(* Logix 5000 AddOnInstructionDefinition export AOI_spLink; software revision 36.00 *)

TYPE DUT_NDSN_spLink :   // UDDT that holds the Cyclic and ACyclic data for the SpectraLink.
STRUCT
   b_r_LostComm : BOOL;
   b_r_PLC_CommReadOnly : BOOL;
   b_r_SystemReady : BOOL;   // Pattern Status Word 0 Bit 0
   b_r_Fault : BOOL;   // Pattern Status Word 0 Bit 1
   b_r_Alert : BOOL;   // Pattern Status Word 0 Bit 2
   b_r_Commissioned : BOOL;   // Pattern Status Word 0 Bit 3
   b_r_RecipeModified : BOOL;   // Pattern Status Word 0 Bit 5
   i_r_Recipe : INT;
   i_r_PalletizedCount : INT;
   i_r_PalletizedSkipCount : INT;
   di_r_App_Trig_ProductCount : DINT;
   di_r_FeedCount : DINT;
   di_r_DeliveryCount : DINT;
   st_r_AppStat : DUT_NDSN_spLink_Chan_Status[8];
   st_r_TrigStat : DUT_NDSN_spLink_Trig_Status[8];
   st_r_EncoStat : DUT_NDSN_spLink_Encoder_Status[8];
   i_r_ProductLength : DINT[8];
   i_r_ProdRate : INT;
   i_r_LineSpeed : INT[2];   // m/min units
   i_r_RunupOutput : INT[2];
   b_w_UnitEnable : BOOL;   // Pattern Control Word 0 Bit 0
   b_w_ClearAllAlarms : BOOL;   // Clear all System Faults and Alerts (Rising Edge).
   b_w_ResetAllCounters : BOOL;   // Reset all counters (rising edge).
   i_w_LoadRecipe : INT;
   i_w_PalletizedCount : INT;   // Write 0 to decrement; 1 to increment; 2 to reset; else does nothing.
   i_w_PalletizedSkipCount : INT;   // Write 0 to decrement; 1 to increment; 2 to reset; else does nothing.
   di_w_App_Trig_ProductCount : DINT;
   di_w_FeedCountReset : DINT;
   di_w_DeliveryCountReset : DINT;
   st_w_AppCtl : DUT_NDSN_spLink_Chan_CTL[8];
   st_rw_BeadAgg : DUT_NDSN_spLink_Bead[8];
   i_rw_RnUpPercentOutP1 : INT[2];
   i_rw_RnUpLineSpdP1 : INT[2];
   i_rw_RnUpPercentOutP2 : INT[2];
   i_rw_RnUpLineSpdP2 : INT[2];
   i_rw_RnUpLowLim : INT[2];
   i_rw_RnUpHighLim : INT[2];
   di_rw_EncoderRes : DINT[2];
   i_rw_TriggerMaskDist : DINT[8];
   i_rw_TriggerChCtl : INT[8];
   i_rw_EncoderChCtl : INT[2];
   i_rw_RandAdjStart : INT[8];
   i_rw_RandAdjEnd : INT[8];
   i_rw_VirtualTriggerSize : DINT[8];
   i_rw_ContStartSpeed : INT[8];
   i_rw_ContStopSpeed : INT[8];
   i_rw_ContKnifeCutDelay : DINT[8];
   i_rw_ContKnifeCutGap : DINT[8];
   di_rw_GTO : DINT[8];
   i_r_ErrorInfo : INT[4];
   i_r_SpecCtl : INT[4];
   i_r_CurrentFault : INT;
END_STRUCT
END_TYPE

TYPE DUT_NDSN_spLink_Bead :
STRUCT
   di_rw_NumOfBeads : DINT;
   di_rw_BeadDelay : DINT[8];   // 1/4 mm
   di_rw_BeadDuration : DINT[8];   // 1/4 mm
   di_rw_mode : DINT;   // 1/4 mm
   di_rw_MaxGunTime : DINT;   // microseconds
   di_rw_LineSpeedActivation : DINT;   // 100th m/min
   di_rw_LineSpeedDeactivation : DINT;   // 100th m/min
   di_rw_Interval : DINT;   // 1/4 mm
   di_rw_AdhesiveSavings : DINT;   // 30%-60%
   di_rw_EcoBeadPattern : DINT;   // 0-40, Illegal values: 0,1,11,20,21,30,31,38,39
END_STRUCT
END_TYPE

TYPE DUT_NDSN_spLink_Chan_CTL :
STRUCT
   b_w_Enable : BOOL;
   b_w_Purge : BOOL;
END_STRUCT
END_TYPE

TYPE DUT_NDSN_spLink_Chan_Status :
STRUCT
   b_r_Enabled : BOOL;
   b_r_Fault : BOOL;
   b_r_Alert : BOOL;
   b_r_Output_Active : BOOL;
   b_r_Installed : BOOL;
END_STRUCT
END_TYPE

TYPE DUT_NDSN_spLink_Encoder_Status :   // SpectraLink Encoder Channel Status
STRUCT
   b_r_Missing : BOOL;
   b_r_Phase_Missing : BOOL;
   b_r_Scaled : BOOL;
   b_r_Fault : BOOL;
   b_r_Alert : BOOL;
   b_r_Installed : BOOL;
END_STRUCT
END_TYPE

TYPE DUT_NDSN_spLink_Rd_Wt :
STRUCT
   i_arr_ReadValue : INT[60];
   i_ReadADI : INT;
   b_ReadDone : BOOL;
   i_arr_WriteValue : INT[60];
   i_WriteADI : INT;
   i_WriteSizeBytes : INT;
   b_WriteEvent : BOOL;
   b_WriteDone : BOOL;
   b_FirstScan : BOOL;
   b_AllowWrites : BOOL;
   b_WriteErr : BOOL;
   b_ReadErr : BOOL;
END_STRUCT
END_TYPE

TYPE DUT_NDSN_spLink_Trig_Status :   // SpectraLink Trigger Channel Status
STRUCT
   b_r_Detected : BOOL;
   b_r_Fault : BOOL;
   b_r_Alert : BOOL;
   b_r_Active : BOOL;
   b_r_Installed : BOOL;
END_STRUCT
END_TYPE

TYPE DUT_spLink_ADI :
STRUCT
   i_ADI : INT;
   i_Size : INT;
END_STRUCT
END_TYPE

ADD_ON_INSTRUCTION AOI_spLink   (* revision 1.0 *)
// AOI to handle the I/O based data (Default Data) and Acyclic Data (low Priority) from the SpectraLink Pattern Controller.
VAR_IN_OUT
   IO_Input : INT[64]; {required}
   IO_Out : INT[64]; {required}
   spLink_HMI : DUT_NDSN_spLink; {required}
   IO_AcycRdWt : DUT_NDSN_spLink_Rd_Wt; {required}
   ReadMsg : MESSAGE; {required}
   WriteMsg : MESSAGE; {required}
   Read_Buffer : INT[100]; {required}
   Write_Buffer : INT[100]; {required}
END_VAR
VAR
   st_ADI_List : DUT_spLink_ADI[40]; {access None}
   tm_Command : FBD_TIMER; {access None}
   tm_Acyc : FBD_TIMER; {access None}
   b_AdhesiveOn : BOOL; {access None}
   b_AdhesiveOff : BOOL; {access None}
   b_Read : BOOL; {access None}
   i_ADI_Range : INT; {access None}
   i_ADI_Size : INT := 20; {access None}
   i_CompareIndex : INT; {access None}
   i_Index : INT; {access None}
   i_Index_Write : INT; {access None}
   i_rwADI_Count : INT := 12; {access None}
   i_rwDataSize : INT := 24; {access None}
   i_Size : INT; {access None}
   i_SizeofStruct : INT := 48; {access None}
   i_ValueIndex : INT; {access None}
   i : INT; {access None}
   i_temp_CPC : INT; {access None}
   arr_WriteIndex : DINT[40]; {access None}
   arr_WriteStartingAddress : DINT[40]; {access None}
   b_AcycWT_Rising : BOOL; {access None}
   arr_HMI : INT[600]; {access None}
   arr_HMI_Buffer : INT[600]; {access None}
   arr_HMI_Compare : INT[600]; {access None}
   b_AcycRD_Rising : BOOL; {access None}
   b_CommandRising : BOOL; {access None}
   tm_PalletizedCount_Reset : FBD_TIMER; {access None}
   b_ResetCurrentPalletizedCount : BOOL; {access None}
   b_ResetCurrentPalletizedSkipCount : BOOL; {access None}
   tm_PalletizedSkipCount_Reset : FBD_TIMER; {access None}
   i_temp_CPSC : INT; {access None}
   i_LoopCnt : INT; {access None}
   b_ResetSelectCount : BOOL; {access None}
   tm_ResetSelectCount : FBD_TIMER := (PRE := 5000); {access None}
   TRUE : BOOL := 1; {access None}
   FALSE : BOOL; {access None}
   tm_ResetFeedCount : FBD_TIMER; {access None}
   tm_ResetDeliveryCount : FBD_TIMER; {access None}
   i_WriteSizeTemp : INT; {access None}
   i_ReadADI_Temp : INT; {access None}
   tm_WriteEvent : FBD_TIMER; {access None}
   b_WriteEventONS : BOOL; {access None}
   i_WritePtr : DINT; {access None}
   Read_Watchdog : FBD_TIMER; {access None}
   Read_Time_Tic : FBD_TIMER; {access None}
   DINT_TEMP : DINT; {access None}
   DINT_Offset : INT; {access Read Only}
END_VAR

ROUTINE Logic   (* structured text *)
   //
   //		SpectraLink Add-On Instruction used to read/write Cyclic (high priority I/O)
   //		and Acyclic (low priority) data.
   //
   //
   //*******************************************************************************
   //	Initialize Code
   //*******************************************************************************
   
   IF IO_AcycRdWt.b_FirstScan THEN
   	i_ADI_Size:= 29;
   	i_rwADI_Count :=26;
   	i_SizeofStruct := 531;
   	i_rwDataSize := 522;
   	i_ADI_Range := 0;
   	i_ValueIndex :=0;
   	i_Index:=0;
   	IO_AcycRdWt.b_FirstScan := 0;		//Reset the FirstScan bit sent to the ADI from the main routine.
   	IO_AcycRdWt.b_AllowWrites := 0;		//Cycle through the full Read Data Set before allowing Writes to occur.  This populates the write compare buffers.
   
   	FOR i := 0 TO i_rwADI_Count DO
   		i_ADI_Range := i_ADI_Range + st_ADI_List[i].i_Size;
   		arr_WriteIndex[i] := i_ADI_Range;					//Index of all Read/Write ADI
   		arr_WriteStartingAddress[i + 1] := i_ADI_Range;		//All Read/Write ADI Starting Address
   	END_FOR;
   
   
   END_IF;
   
   
   
   
   //*******************************************************************************
   //  Start of Cyclic Data Code
   //
   //	The following code handles the I/O data for the High Priority DEFAULT ADIs.
   //*******************************************************************************
   
   // SpectraLink system Status
   spLink_HMI.b_r_SystemReady := IO_Input[0].0;
   spLink_HMI.b_r_Fault := IO_Input[0].1;
   spLink_HMI.b_r_Alert := IO_Input[0].2;
   spLink_HMI.b_r_Commissioned := IO_Input[0].3;
   spLink_HMI.b_r_PLC_CommReadOnly := IO_Input[0].4;
   spLink_HMI.b_r_RecipeModified := IO_Input[0].5;
   
   spLink_HMI.i_r_Recipe := IO_Input[4];
   spLink_HMI.i_r_PalletizedCount := IO_Input[5];
   spLink_HMI.i_r_PalletizedSkipCount := IO_Input[6];
   
   COP(IO_Input[7], spLink_HMI.di_r_App_Trig_ProductCount, 6);
   
   // Copy the Applicator Status Structure Bits from the IO_Inputs
   i_LoopCnt := 0;
   While (i_LoopCnt < 8) DO
   	spLink_HMI.st_r_AppStat[i_LoopCnt].b_r_Enabled := IO_Input[13+i_LoopCnt].0;
   	spLink_HMI.st_r_AppStat[i_LoopCnt].b_r_Fault := IO_Input[13+i_LoopCnt].1;
   	spLink_HMI.st_r_AppStat[i_LoopCnt].b_r_Alert := IO_Input[13+i_LoopCnt].2;
   	spLink_HMI.st_r_AppStat[i_LoopCnt].b_r_Output_Active := IO_Input[13+i_LoopCnt].3;
   	spLink_HMI.st_r_AppStat[i_LoopCnt].b_r_Installed := IO_Input[13+i_LoopCnt].4;
   	i_LoopCnt := i_LoopCnt+1;
   end_while;
   
   // Copy the Trigger Status Structure Bits from the IO_Inputs
   i_LoopCnt := 0;
   While (i_LoopCnt < 8) DO
   	spLink_HMI.st_r_TrigStat[i_LoopCnt].b_r_Detected := IO_Input[21+i_LoopCnt].0;
   	spLink_HMI.st_r_TrigStat[i_LoopCnt].b_r_Fault := IO_Input[21+i_LoopCnt].1;
   	spLink_HMI.st_r_TrigStat[i_LoopCnt].b_r_Alert := IO_Input[21+i_LoopCnt].2;
   	spLink_HMI.st_r_TrigStat[i_LoopCnt].b_r_Active := IO_Input[21+i_LoopCnt].3;
   	i_LoopCnt := i_LoopCnt+1;
   end_while;
   
   // Copy the Encoder Status Structure Bits from the IO_Inputs
   i_LoopCnt := 0;
   While (i_LoopCnt < 2) DO
   	spLink_HMI.st_r_EncoStat[i_LoopCnt].b_r_Missing := IO_Input[29+i_LoopCnt].0;
   	spLink_HMI.st_r_EncoStat[i_LoopCnt].b_r_Phase_Missing := IO_Input[29+i_LoopCnt].1;
   	spLink_HMI.st_r_EncoStat[i_LoopCnt].b_r_Scaled := IO_Input[29+i_LoopCnt].2;
   	spLink_HMI.st_r_EncoStat[i_LoopCnt].b_r_Fault := IO_Input[29+i_LoopCnt].3;
   	spLink_HMI.st_r_EncoStat[i_LoopCnt].b_r_Alert := IO_Input[29+i_LoopCnt].4;
   	i_LoopCnt := i_LoopCnt+1;
   end_while;
   
   
   //******************************************************************************************************************
   //Adjust the Product Length by a factor of 4
   //******************************************************************************************************************
   
   i_LoopCnt := 0;
   While (i_LoopCnt < 8) DO
   	DINT_Offset := i_LoopCnt*2;
   	COP(IO_Input[31+DINT_Offset], DINT_TEMP, 2);
   	spLink_HMI.i_r_ProductLength[i_LoopCnt] := (DINT_TEMP/4);
   	i_LoopCnt := i_LoopCnt+1;
   end_while;
   
   
   COP(IO_Input[47], spLink_HMI.i_r_ProdRate, 1);
   COP(IO_Input[48], spLink_HMI.i_r_LineSpeed[0], 2);
   COP(IO_Input[50], spLink_HMI.i_r_RunupOutput[0], 2);
   
   
   //******************************************************************************************************************
   //Cyclic WRITE Section
   //******************************************************************************************************************
   
   IO_Out[0].0 := spLink_HMI.b_w_UnitEnable;
   IO_Out[2].0 := spLink_HMI.b_w_ClearAllAlarms;
   IO_Out[2].1 := spLink_HMI.b_w_ResetAllCounters;
   
   IO_Out[4] := spLink_HMI.i_w_LoadRecipe;
   
   
   //********************************************************************************************************************************
   //Current Palatized Count & Current Palatized Skip Count     increment (1) or decrement (0);  else = other value     (ADI 16359 Write)
   //********************************************************************************************************************************
   //*********************************************************************
   //PLC logic will set the increment flag (1) or the decrement flag (0) which will generate a 1 second pulse to the spLink.  The
   //command must be set to a "else value" before another increment or decrement can occur.
   //*********************************************************************
   
   IF (spLink_HMI.i_w_PalletizedCount <> i_temp_CPC) AND NOT tm_PalletizedCount_Reset.EN AND NOT b_ResetCurrentPalletizedCount then
   	b_ResetCurrentPalletizedCount := 1;
   	i_temp_CPC := spLink_HMI.i_w_PalletizedCount;
   	tm_PalletizedCount_Reset.Reset := NOT b_ResetCurrentPalletizedCount;
   end_if;
   
   tm_PalletizedCount_Reset.PRE :=2000;
   tm_PalletizedCount_Reset.TimerEnable := b_ResetCurrentPalletizedCount;
   TONR(tm_PalletizedCount_Reset);
   
   If tm_PalletizedCount_Reset.DN then
   	b_ResetCurrentPalletizedCount := 0;
   end_if;
   
   
   IF (tm_PalletizedCount_Reset.EN AND NOT tm_PalletizedCount_Reset.DN AND (i_temp_CPC = 0)) then
   	IO_Out[5] := 0;
   elsif (tm_PalletizedCount_Reset.EN AND NOT tm_PalletizedCount_Reset.DN AND (i_temp_CPC = 1)) then
   	IO_Out[5] := 1;
   else
   	IO_Out[5] := 5;  // anything but a 1 or 0
   end_if;
   
   
   IF (spLink_HMI.i_w_PalletizedSkipCount <> i_temp_CPSC) AND NOT tm_PalletizedSkipCount_Reset.EN AND NOT b_ResetCurrentPalletizedSkipCount then
   	b_ResetCurrentPalletizedSkipCount := 1;
   	i_temp_CPSC := spLink_HMI.i_w_PalletizedSkipCount;
   	tm_PalletizedCount_Reset.Reset := NOT b_ResetCurrentPalletizedSkipCount;
   end_if;
   
   tm_PalletizedSkipCount_Reset.PRE :=2000;
   tm_PalletizedSkipCount_Reset.TimerEnable := b_ResetCurrentPalletizedSkipCount;
   TONR(tm_PalletizedSkipCount_Reset);
   
   IF (tm_PalletizedSkipCount_Reset.EN AND NOT tm_PalletizedSkipCount_Reset.DN AND (i_temp_CPSC = 0)) then
   	IO_Out[6] := 0;
   elsif (tm_PalletizedSkipCount_Reset.EN AND NOT tm_PalletizedSkipCount_Reset.DN AND (i_temp_CPSC = 1)) then
   	IO_Out[6] := 1;
   else
   	IO_Out[6] := 5;  // anything but a 1 or 0
   end_if;
   
   
   If tm_PalletizedSkipCount_Reset.DN then
   	b_ResetCurrentPalletizedSkipCount := 0;
   end_if;
   
   
   //********************************************************************************************************************************
   //Display Select Count, Feed Count and Delivery Count Reset     reset (1) or do nothing (0);        (ADI 16656 Write)
   //********************************************************************************************************************************
   //*********************************************************************
   //PLC logic will set the Reset (1) which will generate a 1 second pulse to the spLink.  The
   //command must be set to a "0" before another Reset can occur.
   //*********************************************************************
   
   
   	tm_ResetSelectCount.PRE := 1000;
   	tm_ResetSelectCount.TimerEnable := spLink_HMI.di_w_App_Trig_ProductCount.0;
   	tm_ResetSelectCount.Reset := NOT spLink_HMI.di_w_App_Trig_ProductCount.0;
   	TONR(tm_ResetSelectCount);
   
   	IF tm_ResetSelectCount.TT then
   		IO_Out[7] := 1;
   	else
   		IO_Out[7] := 0;
   	end_if;
   
   
   	tm_ResetFeedCount.PRE := 1000;
   	tm_ResetFeedCount.TimerEnable := spLink_HMI.di_w_FeedCountReset.0;
   	tm_ResetFeedCount.Reset := NOT spLink_HMI.di_w_FeedCountReset.0;
   	TONR(tm_ResetFeedCount);
   
   	IF tm_ResetFeedCount.TT then
   		IO_Out[9] := 1;
   	else
   		IO_Out[9] := 0;
   	end_if;
   
   
   	tm_ResetDeliveryCount.PRE := 1000;
   	tm_ResetDeliveryCount.TimerEnable := spLink_HMI.di_w_DeliveryCountReset.0;
   	tm_ResetDeliveryCount.Reset := NOT spLink_HMI.di_w_DeliveryCountReset.0;
   	TONR(tm_ResetDeliveryCount);
   
   	IF tm_ResetDeliveryCount.TT then
   		IO_Out[11] := 1;
   	else
   		IO_Out[11] := 0;
   	end_if;
   
   
   //********************************************************************************************************************************
   //Send the Applicator Channel Control Aggregate data to the PC.       (ADI 18675 Write)
   //********************************************************************************************************************************
   
   	i_LoopCnt := 0;
   While (i_LoopCnt < 8) DO
   	IO_Out[13+i_LoopCnt].0 := spLink_HMI.st_w_AppCtl[i_LoopCnt].b_w_Enable;
   	IO_Out[13+i_LoopCnt].1 := spLink_HMI.st_w_AppCtl[i_LoopCnt].b_w_Purge;
   	i_LoopCnt := i_LoopCnt+1;
   end_while;
   
   
   //*******************************************************************************************************************************
   //  Start of Acyclic Data Code
   //
   //	The following code handles the Explicit Messages for the Lower Priority ADIs.
   //*******************************************************************************
   
   tm_Acyc.PRE :=350;
   tm_Acyc.TimerEnable := NOT b_Read AND NOT IO_AcycRdWt.b_WriteEvent;
   TONR(tm_Acyc);
   b_Read :=tm_Acyc.DN;
   
   //Read Message Time Tic (25mSec between Reads)
   
   Read_Time_Tic.PRE := 25;
   Read_Time_Tic.TimerEnable := NOT Read_Time_Tic.DN;
   TONR(Read_Time_Tic);
   
   
   //Read Message Watchdog
   
   Read_Watchdog.PRE :=500;
   Read_Watchdog.TimerEnable := NOT Read_Watchdog.DN;
   TONR(Read_Watchdog);
   Read_Watchdog.Reset := 0;
   
   If Read_Watchdog.DN then
   	i_ReadADI_Temp  := 0;
   
   end_if;
   
   
   //******************************************************************
   //Sequentially read ALL ADIs and store into structure
   //b_read will initiate when tm_Acyc Expired,b_AcycRD_Tick will
   //trigger the funciton block when read is done,
   //b_AcycRD_Enable only last during Acyclic reading in process
   //When last ADI been read, it will stop reading until next cycle
   //*******************************************************************
   IO_AcycRdWt.i_ReadADI := st_ADI_List[i_Index].i_ADI;
   i_Size := st_ADI_List[i_Index].i_Size;
   
   
   If (IO_AcycRdWt.i_ReadADI <> i_ReadADI_Temp) AND Read_Time_Tic.DN then
   
   	ReadMsg.Instance := IO_AcycRdWt.i_ReadADI;
   	MSG(ReadMsg);
   	i_ReadADI_Temp := IO_AcycRdWt.i_ReadADI;
   
   end_if;
   
   IO_AcycRdWt.b_ReadDone := ReadMsg.DN;
   IO_AcycRdWt.b_ReadErr := ReadMsg.ER;
   
   IF IO_AcycRdWt.b_ReadDone AND NOT IO_AcycRdWt.b_WriteEvent AND b_AcycRD_Rising THEN
   
   	COP(Read_Buffer[0],arr_HMI[i_ValueIndex],i_Size);
   
   	//****************************************************
   	//After reading the current ADI, index to next one
   	//****************************************************
   	i_ValueIndex := i_ValueIndex + st_ADI_List[i_Index].i_Size;
       i_Index := i_Index + 1;
   
   	Read_Watchdog.Reset := 1;
   
   END_IF;
   
   b_AcycRD_Rising := NOT IO_AcycRdWt.b_ReadDone;
   
   
   //****************************************************
   //Copy all reading value into structure
   //****************************************************
   IF b_Read THEN
   	COP(arr_HMI[0],spLink_HMI.st_rw_BeadAgg[0],i_SizeofStruct);
   	COP(arr_HMI[0],arr_HMI_Buffer[0],i_rwDataSize);
   END_IF;
   
   IF ((i_Index = i_ADI_Size) AND b_Read) THEN
       i_Index := 0;
   	i_ValueIndex :=0;
   	IO_AcycRdWt.b_AllowWrites := 1;
   END_IF;
   
   //**********************************************************************************************
   //Copy all read/write ADI reading into arr_HMI_Buffer_Compare for further generating Write Event
   //***********************************************************************************************
   COP(spLink_HMI.st_rw_BeadAgg[0],arr_HMI_Compare[0],i_rwDataSize);
   
   //**************************************************************************************
   //Compare arr_HMI_Compare with arr_HMI_Buffer to generate write event
   //**************************************************************************************
   tm_WriteEvent.PRE :=350;
   tm_WriteEvent.TimerEnable :=IO_AcycRdWt.b_WriteEvent;
   TONR(tm_WriteEvent);
   
   
   b_WriteEventONS := 0;
   
   FOR i:=0 TO i_rwDataSize-1 BY 1 DO
   	IF (arr_HMI_Compare[i] <> arr_HMI_Buffer[i]) AND NOT IO_AcycRdWt.b_WriteEvent and IO_AcycRdWt.b_AllowWrites THEN
   
   		i_CompareIndex := i;
   		IO_AcycRdWt.b_WriteEvent := 1;
   		b_WriteEventONS := 1;
   		arr_HMI_Buffer[i] :=arr_HMI_Compare[i];
   
   		EXIT;
   	END_IF;
   END_FOR;
   
   IF b_WriteEventONS THEN
   	//***************************************************************
   	//When write event locate the write index inside arr_WriteIndex
   	//***************************************************************
       FOR i := 0 TO i_rwADI_Count DO
           IF i_CompareIndex < arr_WriteIndex[i] THEN
               i_Index_Write := i;
               EXIT;
           END_IF;
       END_FOR;
   
   	i_WriteSizeTemp := st_ADI_List[i_Index_Write].i_Size;
   	IO_AcycRdWt.i_WriteADI := st_ADI_List[i_Index_Write].i_ADI;
   
   	i_WritePtr := arr_WriteStartingAddress[i_Index_Write];
   	COP(arr_HMI_Compare[i_WritePtr],IO_AcycRdWt.i_arr_WriteValue[0],i_WriteSizeTemp);
   	COP(arr_HMI_Compare[i_WritePtr],arr_HMI[i_WritePtr],i_WriteSizeTemp);
   
   	IO_AcycRdWt.i_WriteSizeBytes := i_WriteSizeTemp*2;
   
   	COP(arr_HMI_Compare[i_WritePtr], Write_Buffer[0],i_WriteSizeTemp);
   	WriteMsg.Instance := IO_AcycRdWt.i_WriteADI;
   	WriteMsg.REQ_LEN := IO_AcycRdWt.i_WriteSizeBytes;
   	MSG(WriteMsg);
   
   END_IF;
   
   	IO_AcycRdWt.b_WriteDone := WriteMsg.DN;
   	IO_AcycRdWt.b_WriteErr := WriteMsg.ER;
   
   IF tm_WriteEvent.DN OR (IO_AcycRdWt.b_WriteDone AND b_AcycWT_Rising) THEN
   	IO_AcycRdWt.b_WriteEvent :=0;
   END_IF;
   b_AcycWT_Rising := NOT IO_AcycRdWt.b_WriteDone;
   
   
   
   
   //
   //   NOTES:  After MSG Write is working, go back and add ERR bits to the IO_AcycRdWt UDDT.
   //
   //
   
   
   
END_ROUTINE
END_ADD_ON_INSTRUCTION
